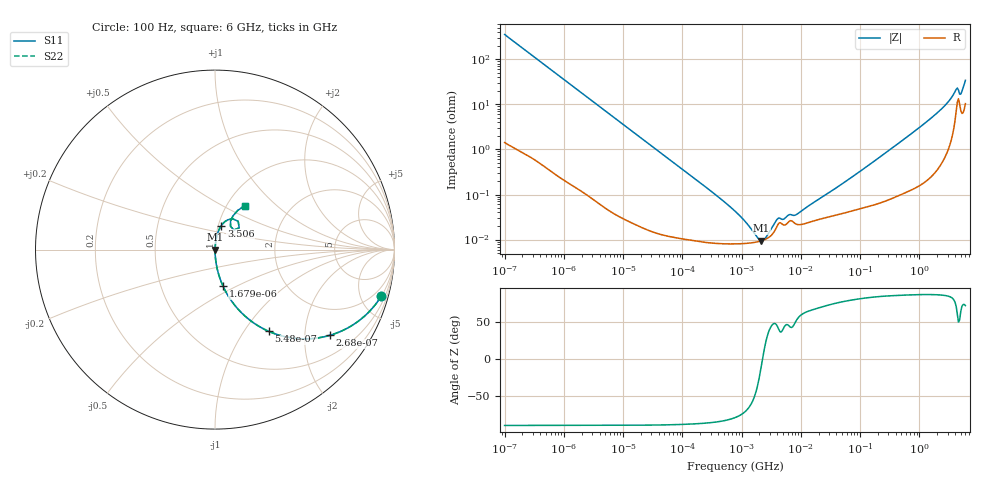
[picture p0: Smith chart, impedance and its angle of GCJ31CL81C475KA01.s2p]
!Murata Part Number: GCJ31CL81C475KA01
!These Parameters are Measured in Series Mode Connection
!Data Generated on Mar 13, 2026
!  o--ll--o
!Port1  Port2
!  o------o
!Operation Temp=25[degC], DC Bias Voltage=0[V]
!Freq. Start=100[Hz] Stop=6[GHz] 401[Steps]
# Hz S RI R 50
!Freq.(Hz) S11(Real) S11(Imag) S21(Real) S21(Imag) S12(Real) S12(Imag) S22(Real) S22(Imag)
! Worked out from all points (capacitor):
!   401 points, 100 Hz to 6 GHz, reference 50 ohm
!   read as one part in series: C = 4.47 uF near 109 Hz
!   lowest |Z| = 9.49 mohm at 2.169 MHz (marker M1)
!   series resonance near 2.259 MHz, so ESL is about 1.1 nH
!   S11 on the Smith chart (normalised r, x): 100 Hz: 1.03, -7.11; 268 Hz: 1.01, -2.66; 548 Hz: 1.01, -1.30; 1.679 kHz: 1.00, -0.43; 3.506 GHz: 1.03, +0.28; 6 GHz: 1.21, +0.65
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100  0.9258 -0.2601  0.0742 0.2601  0.0742 0.2601  0.9258 -0.2601
164  0.8244 -0.3782  0.1756 0.3782  0.1756 0.3782  0.8244 -0.3782
268  0.6386 -0.4778  0.3614 0.4778  0.3614 0.4778  0.6386 -0.4778
548  0.2994 -0.4552  0.7006 0.4552  0.7006 0.4552  0.2994 -0.4552
938  0.1286 -0.3319  0.8714 0.3319  0.8714 0.3319  0.1286 -0.3319
1679  0.0449 -0.2039  0.9551 0.2039  0.9551 0.2039  0.0449 -0.2039
2008  0.032 -0.1729  0.968 0.1729  0.968 0.1729  0.032 -0.1729
6433  0.00353 -0.0559  0.9965 0.0559  0.9965 0.0559  0.00353 -0.0559
40335  0.000214 -0.009  0.9998 0.009  0.9998 0.009  0.000214 -0.009
774597  8.03e-05 -0.00042  0.9999 0.00042  0.9999 0.00042  8.03e-05 -0.00042
1813585  8.85e-05 -7.34e-05  0.9999 7.34e-05  0.9999 7.34e-05  8.85e-05 -7.34e-05
2169299  9.39e-05 -1.35e-05  0.9999 1.35e-05  0.9999 1.35e-05  9.39e-05 -1.35e-05
2594782  0.000103 4.76e-05  0.9999 -4.76e-05  0.9999 -4.76e-05  0.000103 4.76e-05
4060267  0.000209 0.0002  0.9998 -0.0002  0.9998 -0.0002  0.000209 0.0002
8311524  0.000221 0.000278  0.9998 -0.000278  0.9998 -0.000278  0.000221 0.000278
1.555665e7  0.000253 0.00058  0.9997 -0.00058  0.9997 -0.00058  0.000253 0.00058
3.124326e8  0.000865 0.00964  0.9991 -0.00964  0.9991 -0.00964  0.000865 0.00964
1.712697e9  0.00561 0.0535  0.9944 -0.0535  0.9944 -0.0535  0.00561 0.0535
3.505958e9  0.0354 0.1339  0.9646 -0.1339  0.9646 -0.1339  0.0354 0.1339
4.193612e9  0.0975 0.1718  0.9025 -0.1718  0.9025 -0.1718  0.0975 0.1718
5.016141e9  0.0865 0.1298  0.9135 -0.1298  0.9135 -0.1298  0.0865 0.1298
6e9  0.1663 0.2456  0.8337 -0.2456  0.8337 -0.2456  0.1663 0.2456
